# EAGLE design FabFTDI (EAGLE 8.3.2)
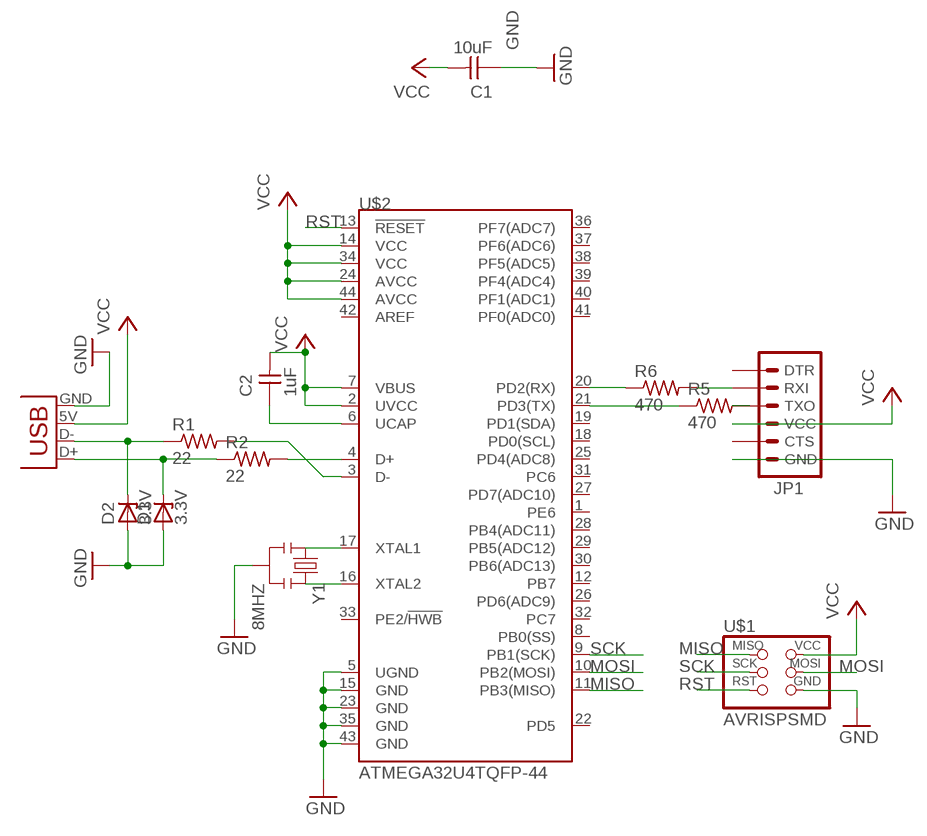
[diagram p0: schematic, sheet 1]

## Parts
C1  10uF  UNPOLARIZED_CAPACITOR1206  [1206]
C2  1uF  UNPOLARIZED_CAPACITOR1206  [1206]
D1  3.3V  ZENER_DIODESOD123  [SOD123]
D2  3.3V  ZENER_DIODESOD123  [SOD123]
JP1  FTDI_CONNECTORSMD  [1X06-SMD]
JP2  USBPCB  [USB_PCB]
R1  22  RESISTOR1206  [1206]
R2  22  RESISTOR1206  [1206]
R5  470  RESISTOR1206  [1206]
R6  470  RESISTOR1206  [1206]
U$1  AVRISPSMD  [2X03SMD]
U$2  ATMEGA32U4TQFP-44  [TQFP44]
Y1  8MHZ  RESONATOR8MHZ  [RESONATOR-SMD]

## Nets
GND: C1.1 D1.ANODE D2.ANODE JP1.6(GND) JP2.GND U$1.6(GND) U$2.5(UGND) U$2.15(GND) U$2.23(GND) U$2.35(GND) U$2.43(GND) Y1.2
MISO: U$1.1(MISO) U$2.11(PB3(MISO))
MOSI: U$1.4(MOSI) U$2.10(PB2(MOSI))
N$1: D1.CATHODE JP2.D+ R2.1
N$2: D2.CATHODE JP2.D- R1.1
N$3: U$2.17(XTAL1) Y1.1
N$4: R1.2 U$2.3(D-)
N$7: JP1.2(RXI) R6.2
N$8: JP1.3(TXO) R5.2
N$9: U$2.16(XTAL2) Y1.3
N$10: R2.2 U$2.4(D+)
N$11: C2.1 U$2.6(UCAP)
N$12: R6.1 U$2.20(PD2(RX))
N$13: R5.1 U$2.21(PD3(TX))
RST: U$1.5(RST) U$2.13(!RESET)
SCK: U$1.3(SCK) U$2.9(PB1(SCK))
VCC: C1.2 C2.2 JP1.4(VCC) JP2.5V(VBUS) U$1.2(VCC) U$2.2(UVCC) U$2.7(VBUS) U$2.14(VCC) U$2.24(AVCC) U$2.34(VCC) U$2.44(AVCC)
Unconnected: JP1.1(DTR) JP1.5(CTS) U$2.1(PE6) U$2.8(PB0(SS)) U$2.12(PB7) U$2.18(PD0(SCL)) U$2.19(PD1(SDA)) U$2.22(PD5) U$2.25(PD4(ADC8)) U$2.26(PD6(ADC9)) U$2.27(PD7(ADC10)) U$2.28(PB4(ADC11)) U$2.29(PB5(ADC12)) U$2.30(PB6(ADC13)) U$2.31(PC6) U$2.32(PC7) U$2.33(PE2/!HWB) U$2.36(PF7(ADC7)) U$2.37(PF6(ADC6)) U$2.38(PF5(ADC5)) U$2.39(PF4(ADC4)) U$2.40(PF1(ADC1)) U$2.41(PF0(ADC0)) U$2.42(AREF)

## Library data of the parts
C1 C2 = fabPatil:UNPOLARIZED_CAPACITOR: unpolarized_capacitor
D1 D2 = fabPatil:ZENER_DIODE: zener diode
JP1 = fabPatil:FTDI_CONNECTOR: FTDI connector smd
JP2 = fabPatil:USB: USB Connector Connector for USB-microB (orAB), USB-mini, and USB-PCB. For USB-micro use Digikey Part# 609-4052-1-ND (typeB) or 609-4052-1-ND (typeAB).
R1 R2 R5 R6 = fabPatil:RESISTOR
U$1 = fabPatil:AVRISP
U$2 = SparkFun-DigitalIC:ATMEGA32U4: Atmel 44-pin 8-bit Microcontroller with 32KBytes of ISP Flash and USB Controller
Y1 = fabPatil:RESONATOR: Resonator Small SMD resonator. Used, eg, on the Arduino Pro/ Pro Mini boards. 8MHz- XTAL-08895 16MHz- XTAL-08900; PROD_ID: XTAL-08895

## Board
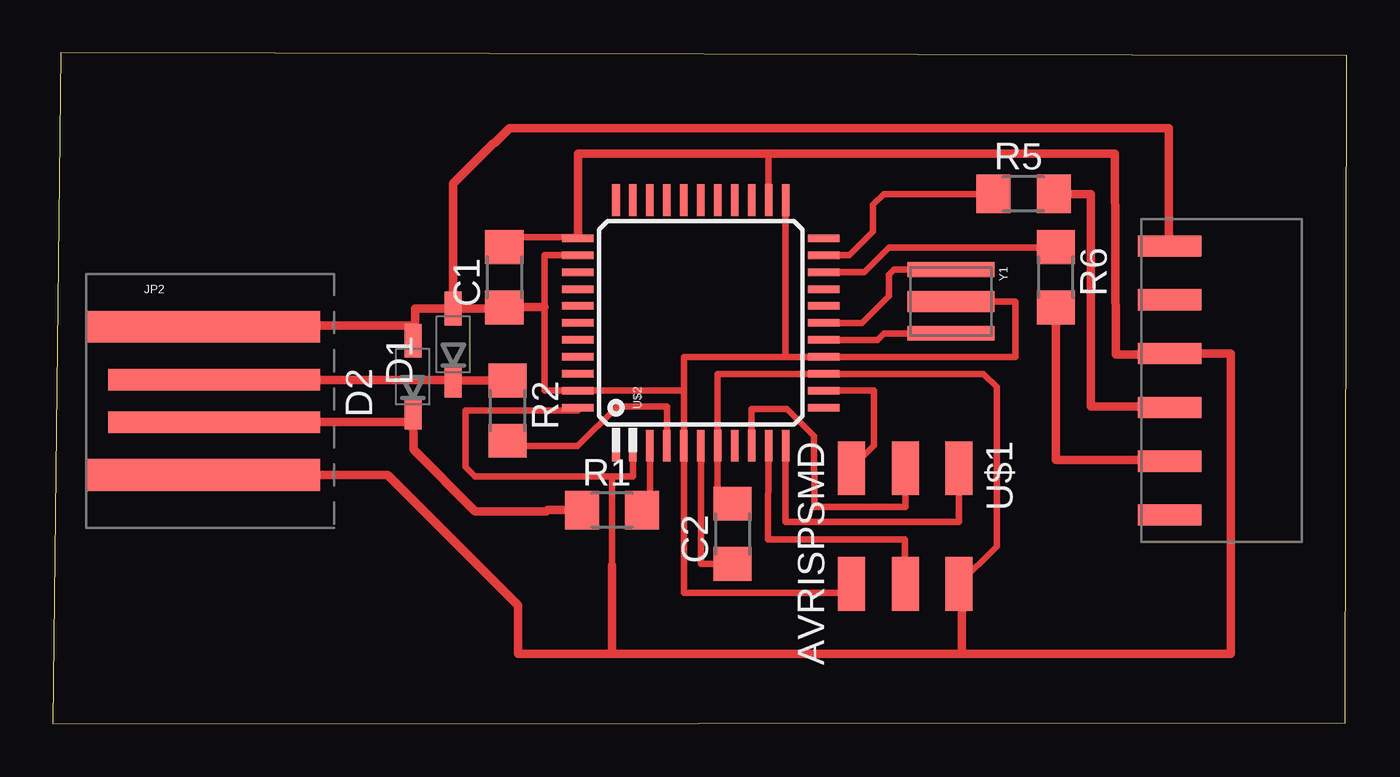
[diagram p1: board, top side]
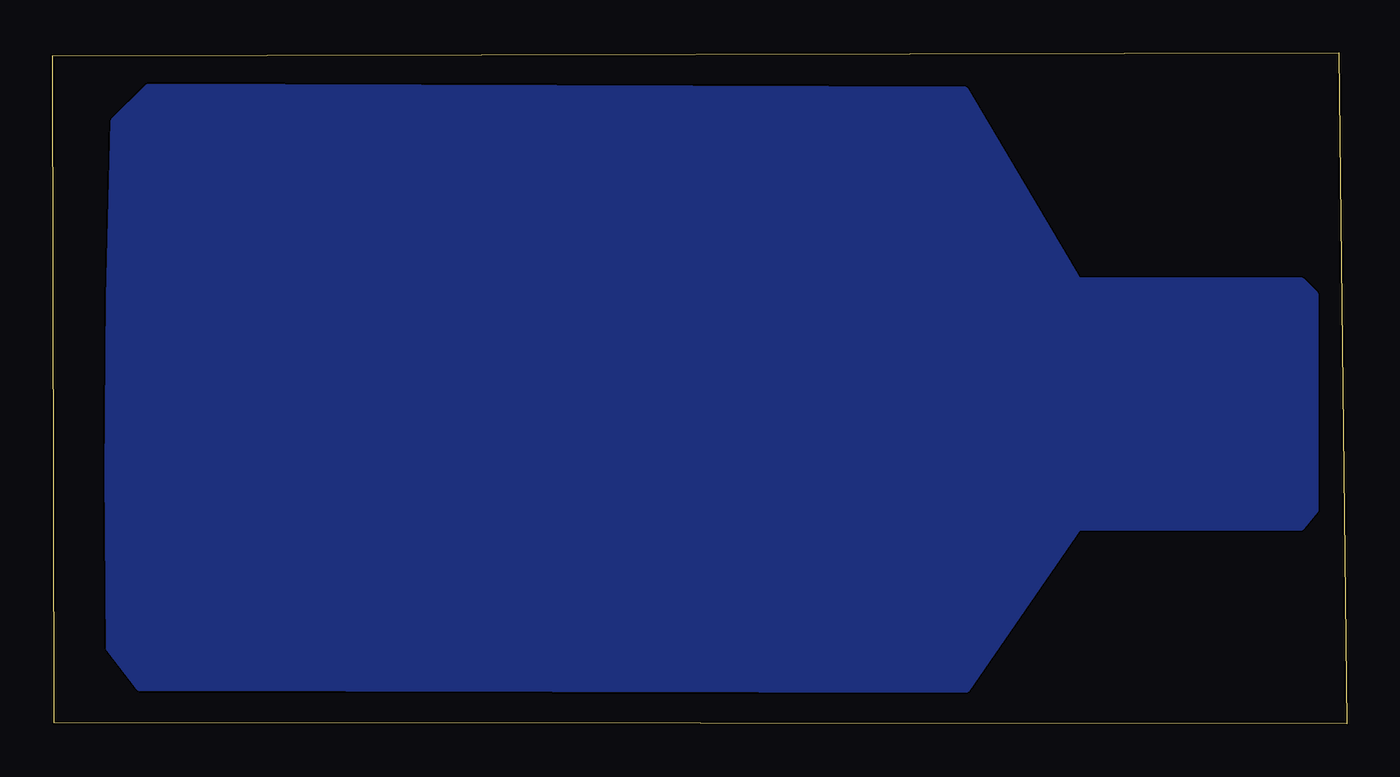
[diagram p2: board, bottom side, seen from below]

Size 61.07 x 31.67 mm. Coordinates in mm from the lower left corner, seen from the top.
Outline: 0,0 61.01,0.05 61.07,31.55 0.36,31.67 0,0
Copper layers (1*16): Top 0.035mm / dielectric 1.5mm / Bottom 0.035mm
Design rules "Patil": minimum track width 10mil, minimum drill 24mil, track to track 16mil, track to pad 16mil, pad to pad 16mil, via to via 16mil, smd to smd 16mil, copper to edge 40mil, drill to drill 8mil, minimum pad ring 10mil, minimum via ring 8mil, stop-mask expansion 4mil, vias tented up to drill 0mil, thermal gap 10mil

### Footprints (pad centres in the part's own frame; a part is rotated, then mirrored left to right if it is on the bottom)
1206 = smd 1.6 x 1.803: 1 -1.422,0; 2 1.422,0
SOD123 = smd 1.6 x 0.8: ANODE 1.7,0; CATHODE -1.7,0
1X06-SMD = smd 1 x 3: 1 -6.35,-1.35; 2 -3.81,-1.35; 3 -1.27,-1.35; 4 1.27,-1.35; 5 3.81,-1.35; 6 6.35,-1.35
USB_PCB = smd 11 x 1.5: 5V 1.55,-3.5; GND 1.55,3.5 | smd 10 x 1: D+ 2.05,1; D- 2.05,-1
2X03SMD = smd 2.54 x 1.27: 1 -2.54,2.54; 2 2.92,2.54; 3 -2.54,0; 4 2.92,0; 5 -2.54,-2.54; 6 2.92,-2.54
TQFP44 = smd 1.499 x 0.356: 1 -5.8,4; 2 -5.8,3.2; 3 -5.8,2.4; 4 -5.8,1.6; 5 -5.8,0.8; 6 -5.8,0; 7 -5.8,-0.8; 8 -5.8,-1.6; 9 -5.8,-2.4; 10 -5.8,-3.2; 11 -5.8,-4; 23 5.8,-4; 24 5.8,-3.2; 25 5.8,-2.4; 26 5.8,-1.6; 27 5.8,-0.8; 28 5.8,0; 29 5.8,0.8; 30 5.8,1.6; 31 5.8,2.4; 32 5.8,3.2; 33 5.8,4 | smd 0.356 x 1.499: 12 -4,-5.8; 13 -3.2,-5.8; 14 -2.4,-5.8; 15 -1.6,-5.8; 16 -0.8,-5.8; 17 0,-5.8; 18 0.8,-5.8; 19 1.6,-5.8; 20 2.4,-5.8; 21 3.2,-5.8; 22 4,-5.8; 34 4,5.8; 35 3.2,5.8; 36 2.4,5.8; 37 1.6,5.8; 38 0.8,5.8; 39 0,5.8; 40 -0.8,5.8; 41 -1.6,5.8; 42 -2.4,5.8; 43 -3.2,5.8; 44 -4,5.8
RESONATOR-SMD = smd 0.7 x 4.1: 1 -1.5,0; 3 1.5,0 | smd 1 x 4.1: 2 0,0

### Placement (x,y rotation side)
C1  21.31,21.08 90 top
C2  32.08,8.97 90 top
D1  18.9,17.91 90 top
D2  16.99,16.38 90 top
JP1  51.36,16.21 90 top
JP2  5.56,15.24 0 top
R1  26.39,10.08 0 top
R2  21.46,14.78 270 top
R5  45.82,25.02 0 top
R6  47.35,21.08 270 top
U$1  40.23,9.53 270 top
U$2  30.58,18.92 90 top
Y1  42.39,19.94 270 top

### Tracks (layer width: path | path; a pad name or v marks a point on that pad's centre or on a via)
GND
  Top 0.305: U$2.23 34.58,17.32 | 34.58,17.32 U$2.15 45.44,17.32 45.44,19.94 Y1.2 | U$2.35 23.22,22.12 23.22,19.68 23.22,15.72 U$2.43 29.78,15.72 | U$1.6 37.69,6.17 29.78,6.17 U$2.5 29.78,15.72 | 29.78,15.72 29.78,17.32 34.58,17.32
  Top 0.406: 17.09,18.19 17.16,18.25 17.16,18.63 arc90 16.99,18.8 7.17,18.8 arc90 JP2.GND | 17.09,18.19 D2.ANODE | D1.ANODE 17.09,19.61 17.09,18.19 | D1.ANODE 21.26,19.61 C1.1 21.31,19.68 23.22,19.68 | D1.ANODE 18.9,25.5 20.8,27.41 20.85,27.41 21.56,28.12 52.68,28.12 52.68,22.58 JP1.6
MISO
  Top 0.305: U$2.11 34.58,9.53 42.77,9.53 U$1.1
MOSI
  Top 0.305: U$1.4 40.21,8.71 33.76,8.71 U$2.10
N$1
  Top 0.406: JP2.D+ 18.9,16.24 D1.CATHODE R2.1
N$2
  Top 0.406: JP2.D- 16.75,14.24 17.12,14.61 17.07,14.61 D2.CATHODE 17.02,12.95 19.94,10.03 23.29,10.03 23.34,10.08 R1.1
N$3
  Top 0.305: U$2.17 38.2,18.92 39.47,20.19 39.47,21.21 39.7,21.44 Y1.1
N$4
  Top 0.305: U$2.3 28.18,10.76 R1.2
N$6
  pour Bottom (no thermals): 1.52,20.24 2.16,20.88 12.7,20.88 18.03,29.9 56.52,30.02 58.14,28.42 arc-3 58.37,3.56 56.97,1.75 17.98,1.65 12.7,9.32 2.16,9.32 1.52,10.08
N$7
  Top 0.406: R6.2 47.35,12.45 52.66,12.45 JP1.2
N$8
  Top 0.406: R5.2 49,25.02 49,14.99 52.66,14.99 JP1.3
N$9
  Top 0.305: U$2.16 38.93,18.12 39.22,18.41 42.37,18.41 Y1.3
N$10
  Top 0.305: U$2.4 28.98,14.99 26.64,14.99 24.77,13.11 21.46,13.11
  Top 0.406: R2.2 21.46,13.11
N$11
  Top 0.305: U$2.6 30.58,7.54 C2.1
N$12
  Top 0.305: R6.1 47.35,22.48 39.47,22.48 38.32,21.32 U$2.20
N$13
  Top 0.305: U$2.21 37.59,22.12 38.71,23.24 38.71,24.51 39.22,25.02 R5.1
RST
  Top 0.305: U$1.5 38.76,13.13 38.76,15.72 | 38.76,15.72 | U$2.13 | U$2.13 38.76,15.72
SCK
  Top 0.305: U$2.9 32.98,14.86 34.66,14.86 35.92,13.6 35.94,10.24 40.23,10.24 U$1.3
VCC
  Top 0.305: U$2.7 31.38,16.52 U$2.14 43.92,16.52 44.55,15.89 44.55,8.38 U$1.2 | U$2.7 31.34,13.12 | U$2.24 33.78,26.92 | 26.4,7.47 26.4,11.24 26.39,11.24 26.39,11.68 | U$2.2 27.38,11.68 26.39,11.68 | 21.79,22.98 24.78,22.98 | U$2.44 24.78,14.78 19.48,14.78 19.48,12.12 19.92,11.68 26.39,11.68 | U$2.7 31.38,11.09 C2.2
  Top 0.406: U$2.34 24.78,22.98 24.78,26.92 33.78,26.92 50.14,26.92 50.16,17.42 52.66,17.42 JP1.4 55.6,17.48 55.6,3.3 42.9,3.3 | JP2.5V 15.79,11.74 21.95,5.59 21.95,3.3 26.4,3.3 | C1.2 21.79,22.98 | 26.4,7.47 26.4,3.3 | 42.9,3.3 26.4,3.3 | U$1.2 42.9,6.61 42.9,3.3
